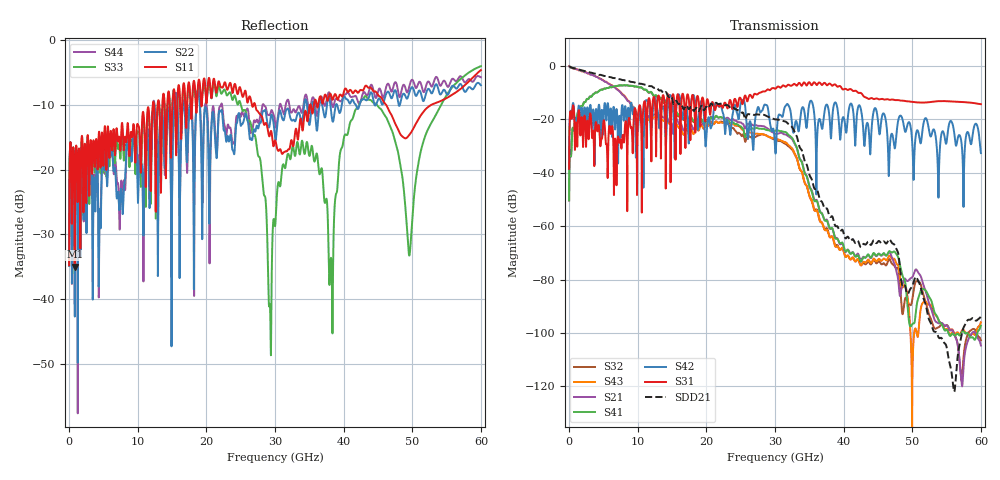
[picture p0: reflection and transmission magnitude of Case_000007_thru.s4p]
! Info: Touchstone file created by circ.  Input file=CasetestDOE_NRZ_template_000007.circ
# Hz S RI R 50
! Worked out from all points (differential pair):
!   6000 points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, 10 MHz to 60 GHz, reference 50 ohm
!   strongest paths, dB at 10 MHz, 15.01 GHz, 30.01 GHz, 45.01 GHz, 60 GHz:
!     S31: -38.5, -11.6, -8.5, -12.4, -14.3
!     S42: -38.5, -13.1, -30.5, -20.6, -32.6
!     S41: -50.4, -14.7, -24.3, -70.5, -97.3
!     S21: -0.1, -22.2, -25.4, -70.6, -104.7
!     S43: -0.1, -22.1, -27.2, -72.5, -96.0
!     S32: -50.4, -15.8, -27.6, -73.3, -102.7
!   taken as a pair (ports 1,3 in; 2,4 out), SDD21 dB: -0.1, -12.0, -20.0, -65.8, -93.8
!   lowest |S11| = -35.0 dB at 830 MHz (marker M1), VSWR 1.04, Z = 51.5 - j0.964 ohm
!   |S11| at or under -10 dB: start of sweep to 12.2 GHz; 27.11 GHz to 35.11 GHz (7.993 GHz wide, 25.7 % of centre); 46.2 GHz to 52.78 GHz (6.576 GHz wide, 13.3 % of centre)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
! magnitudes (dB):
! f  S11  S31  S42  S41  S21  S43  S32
! 10 MHz  -34.7  -38.5  -38.5  -50.4  -0.1  -0.1  -50.4
! 830 MHz  -35.0  -27.4  -23.6  -21.9  -0.9  -0.9  -21.9
! 23.4 GHz  -6.7  -12.9  -24.1  -21.1  -20.1  -21.9  -22.5
! 29.26 GHz  -14.7  -9.1  -21.2  -24.3  -24.1  -26.6  -26.8
! 40.4 GHz  -7.6  -8.7  -24.9  -69.4  -69.4  -71.4  -71.5
! 49.58 GHz  -14.6  -13.3  -21.2  -96.5  -80.0  -93.4  -89.3
! 60 GHz  -4.6  -14.3  -32.6  -97.3  -104.7  -96.0  -102.7
